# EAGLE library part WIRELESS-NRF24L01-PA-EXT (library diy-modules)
2.4 GHz Wireless Module based on NRF24L01 chip with preamplifier and external antenna Click here to find device on ebay.com
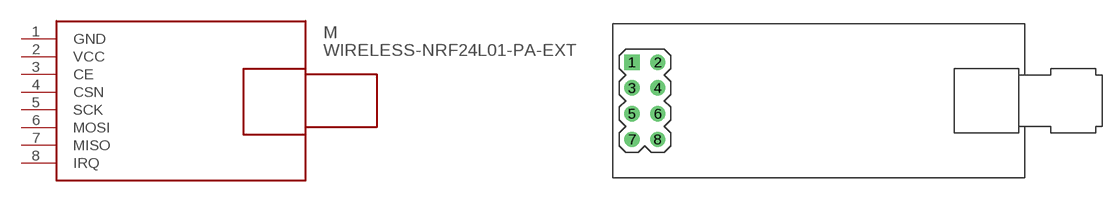
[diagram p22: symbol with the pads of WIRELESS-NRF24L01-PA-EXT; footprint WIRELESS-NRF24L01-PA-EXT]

Designator prefix M

## WIRELESS-NRF24L01-PA-EXT  [WIRELESS-NRF24L01-PA-EXT]
1  GND  pwr
2  VCC  pwr
3  CE
4  CSN
5  SCK
6  MOSI
7  MISO
8  IRQ

## Footprint WIRELESS-NRF24L01-PA-EXT (pad centres in mm)
2.4 GHz Wireless Module based on NRF24L01 chip with preamplifier and external antenna
drill 1 square: 1 -18.415,3.81
drill 1: 2 -15.875,3.81; 3 -18.415,1.27; 4 -15.875,1.27; 5 -18.415,-1.27; 6 -15.875,-1.27; 7 -18.415,-3.81; 8 -15.875,-3.81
